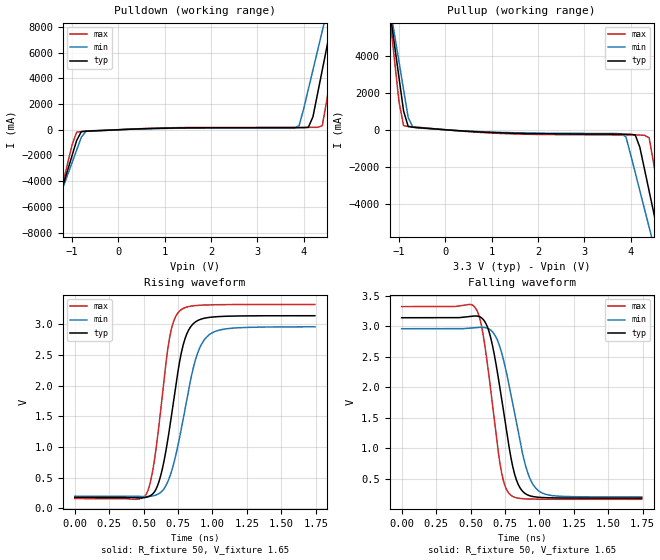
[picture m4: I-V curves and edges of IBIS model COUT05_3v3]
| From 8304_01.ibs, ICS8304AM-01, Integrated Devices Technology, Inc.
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[Model] COUT05_3v3
Model_type   Output
Polarity   Non-Inverting
|   typ   min   max
C_comp   2pF   1.5pF   2.5pF
Vmeas = 1.65V
Rref = 50
Cref = 0
Vref = 1.65V
|   typ   min   max
[Voltage range]   3.3V   3.135V   3.465V
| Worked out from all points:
|   slope of the pulldown table from 0 to 0.495 V, typ, clamps not added: 6.88 ohm
|   slope of the pullup table from 0 to 0.495 V, typ, clamps not added: 5.83 ohm
|   rising waveform, R_fixture 50, V_fixture 1.65: 20-80 % time 127ps typ, 154ps min, 103ps max; typ from 0.181 V to 3.14 V
|   falling waveform, R_fixture 50, V_fixture 1.65: 20-80 % time 128ps typ, 151ps min, 107ps max; typ from 3.14 V to 0.181 V
[Pulldown]
|Voltage   I (typ)   I (min)   I (max)
-3.3V     -29.26A    -25.28A    -35.95A
-1.5V     -7.949A    -7.508A    -8.752A
-900mV    -829.9mA   -1.575A    -187.1mA
-700mV    -111.2mA   -118.1mA   -127.5mA
3.9V      159.4mA    311mA      182.9mA
4.1V      184.8mA    3.152A     184mA
4.2V      1.015A     4.66A      185mA
4.4V      4.637A     7.679A     308.5mA
4.6V      8.262A     10.7A      4.646A
4.7V      10.08A     12.21A     6.964A
4.8V      11.89A     13.72A     9.282A
6.6V      44.81A     41.14A     51.33A
[Pullup]
|Voltage   I (typ)   I (min)   I (max)
-3.3V     44.73A     38.61A     55.03A
-1.2V     6.49A      6.732A     6.202A
-1.1V     4.667A     5.214A     3.875A
-900mV    1.021A     2.176A     220.8mA
-700mV    135.9mA    139mA      157.7mA
3.8V      -238.9mA   -217.3mA   -279.5mA
4.1V      -276.1mA   -2.314A    -283.5mA
4.3V      -2.128A    -4.28A     -299.6mA
4.4V      -3.308A    -5.264A    -428.8mA
4.6V      -5.67A     -7.233A    -3.347A
4.8V      -8.032A    -9.203A    -6.363A
6.6V      -29.3A     -26.93A    -33.51A
[Ramp]
|   typ   min   max
dV/dt_r   2.374/0.197n   2.212/0.24n   2.539/0.159n
dV/dt_f   2.39/0.193n   2.226/0.229n   2.557/0.16n
R_load =   50.0000
[Rising Waveform]
R_fixture = 50
V_fixture = 1.65   |Vcc_typ
V_fixture_min = 1.5675 |Vcc_min
V_fixture_max = 1.7325 |Vcc_max
C_fixture = 0.0p
| Time   typ   min   max
0s        180.7mV    199.5mV    160.8mV
520.5ps   183.7mV    193.6mV    238.7mV
572.6ps   253.4mV    207.2mV    702.8mV
631.1ps   597.9mV    276.8mV    1.746V
696.2ps   1.42V      560mV      2.869V
767.8ps   2.469V     1.228V     3.231V
813.3ps   2.843V     1.767V     3.282V
878.4ps   3.043V     2.438V     3.306V
976ps     3.113V     2.83V      3.317V
1.744ns   3.14V      2.96V      3.323V
[Falling Waveform]
R_fixture = 50
V_fixture = 1.65   |Vcc_typ
V_fixture_min = 1.5675 |Vcc_min
V_fixture_max = 1.7325 |Vcc_max
C_fixture = 0.0p
| Time   typ   min   max
0s        3.141V     2.96V      3.323V
540ps     3.169V     2.979V     3.285V
585.6ps   3.128V     2.983V     2.941V
644.1ps   2.836V     2.942V     2.006V
722.2ps   1.868V     2.597V     639.8mV
793.8ps   843.8mV    1.879V     227.6mV
839.3ps   443.3mV    1.347V     182.7mV
904.4ps   245.1mV    677.6mV    167.6mV
995.5ps   194mV      299.1mV    162.9mV
1.744ns   180.7mV    199.6mV    160.8mV
